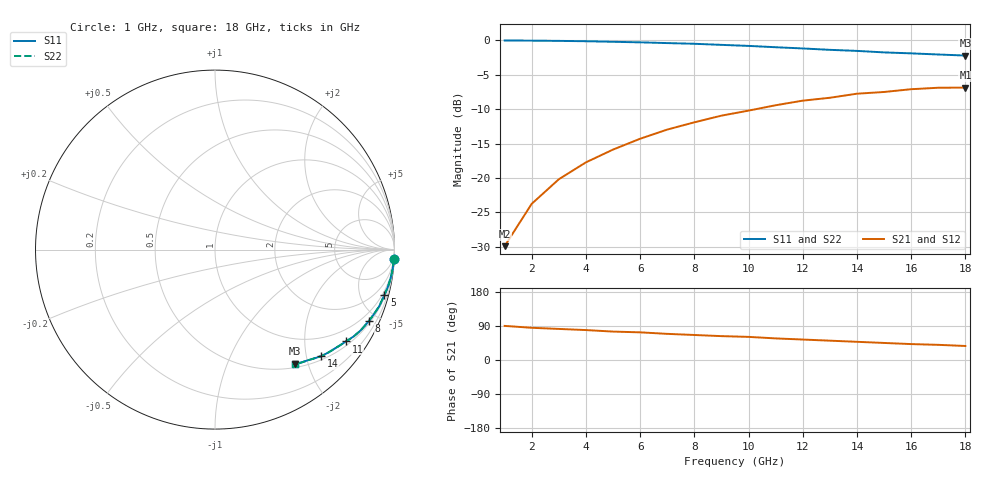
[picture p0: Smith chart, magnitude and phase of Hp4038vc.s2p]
!HPND-4038 beam lead PIN diode
!Series configuration S-parameters Vr= 30 V.  Last updated 10/3/97
# mhz s ma r 50
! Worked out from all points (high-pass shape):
!   18 points, 1 GHz to 18 GHz, reference 50 ohm
!   highest |S21| = -6.86 dB at 18 GHz (marker M1); lowest = -29.9 dB at 1 GHz (marker M2)
!   |S21| within 3 dB of the highest: 10.44 GHz to end of sweep
!   lowest |S11| = -2.2 dB at 18 GHz (marker M3), VSWR 7.93, Z = 27.9 - j89.3 ohm
!   |S11| at or under -10 dB: nowhere
!   |S22| runs from -2.2 to 0.0 dB; largest |S21 - S12| = 0
!   S11 on the Smith chart (normalised r, x): 1 GHz: 1, -38; 5 GHz: 0.68, -7.54; 8 GHz: 0.59, -4.43; 11 GHz: 0.61, -3.06; 14 GHz: 0.57, -2.29; 18 GHz: 0.56, -1.79
1000  0.999 -3.0  0.032 90.0  0.032 90.0  0.999 -3.0
2000  0.996 -6.0  0.065 85.0  0.065 85.0  0.996 -6.0
3000  0.992 -9.0  0.098 82.0  0.098 82.0  0.992 -9.0
4000  0.986 -12.0  0.13 79.0  0.13 79.0  0.986 -12.0
5000  0.977 -15.0  0.161 75.0  0.161 75.0  0.977 -15.0
6000  0.968 -19.0  0.193 73.0  0.193 73.0  0.968 -19.0
7000  0.956 -22.0  0.225 69.0  0.225 69.0  0.956 -22.0
8000  0.945 -25.0  0.254 66.0  0.254 66.0  0.945 -25.0
9000  0.928 -29.0  0.284 63.0  0.284 63.0  0.928 -29.0
10000  0.912 -32.0  0.309 61.0  0.309 61.0  0.912 -32.0
11000  0.892 -35.0  0.338 57.0  0.338 57.0  0.892 -35.0
12000  0.874 -38.0  0.365 54.0  0.365 54.0  0.874 -38.0
13000  0.854 -42.0  0.383 51.0  0.383 51.0  0.854 -42.0
14000  0.839 -45.0  0.41 48.0  0.41 48.0  0.839 -45.0
15000  0.818 -48.0  0.422 45.0  0.422 45.0  0.818 -48.0
16000  0.805 -50.0  0.442 42.0  0.442 42.0  0.805 -50.0
17000  0.79 -53.0  0.453 40.0  0.453 40.0  0.79 -53.0
18000  0.776 -55.0  0.454 37.0  0.454 37.0  0.776 -55.0
